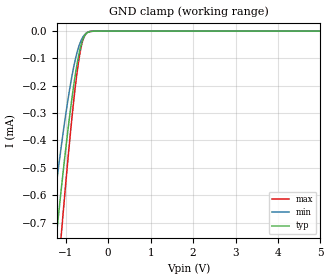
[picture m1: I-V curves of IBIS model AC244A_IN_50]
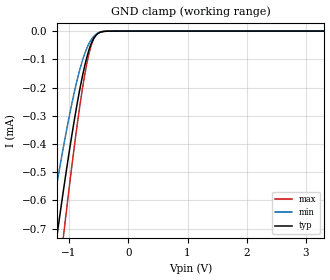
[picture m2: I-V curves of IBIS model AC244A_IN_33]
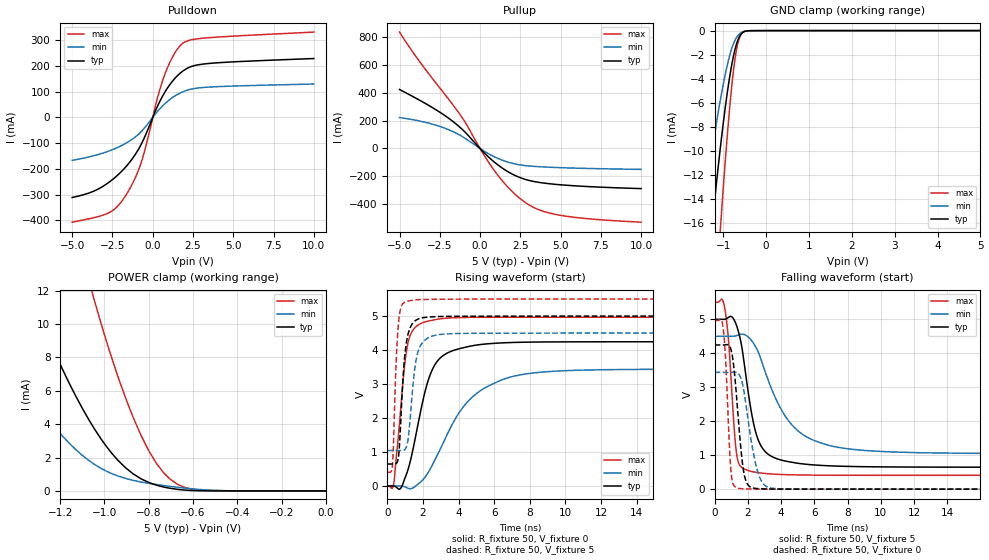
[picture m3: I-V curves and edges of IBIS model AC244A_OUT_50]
| TEXAS INSTRUMENTS INCORPORATED
| Standard Linear and Logic Group
| IBIS Model of SN74AC244
| OCTAL BUFFERS/DRIVERS WITH 3-STATE OUTPUTS
| This file contains package information for the following:
|  TSSOP 20-pin (PW) package as [Component] SN74AC244_PW
| This device can be powered at the following Vccs:
|  5 volt Vcc
|  3.3 volt Vcc
| This file provides unique models under the [Model Selector] for each Vcc.
| For operation at a specific Vcc, select the appropriate model after each
| [Model Selector] keyword.
[IBIS Ver]   3.2
[Comment char]  |_char
[File Name]   sn54ac244.ibs
[File Rev]   1.0 | a_die
[Date]   September 18, 2009
[Source]   Data created from TI-SPICE simulations at TI-SLL.
[Notes]   The following is an IBIS list for the SN74AC244.
   Please contact sllibis@ti.com with questions and
   comments concerning SLL IBIS models.
|   Modified from SN74 to SN54 devices with modified package
|   parasitics.   WVB 091809
[Disclaimer] Property of Texas Instruments Incorporated.  Unauthorized
   reproduction and/or distribution is strictly prohibited.
   This product is protected under copyright law.
   Created  2009, (C) Copyright  2009, Texas Instruments
   Incorporated, All Rights Reserved
   UNLESS THERE IS A SIGNED, WRITTEN AGREEMENT TO THE
   CONTRARY, TEXAS INSTRUMENTS (TI) IS PROVIDING THE IBIS
   MODELS  AND WITHOUT ANY WARRANTY, EXPRESSED OR
   IMPLIED.  TI assumes no liability for:
   1) the accuracy of the IBIS models provided to your
   company;
   2) the proper functioning of these IBIS Models in your
   design or for any resulting applications; or
   3) infringement of patents, copyrights or intellectual
   property rights resulting from your use of these IBIS
   models.
   TI provides IBIS Models as a service to our customers.
   You and your company shall not distribute, sell or give
   these models to anyone else without prior written
   permission from TI.
   TI reserves the right to make changes to our products or
   to discontinue any semiconductor product or service
   without notice, and advises our customers to obtain the
   latest version of relevant information to verify, before
   placing orders, that the information being relied on is
   current.
   Please be aware that your receipt and use of the IBIS
   information provided shall serve as acceptance of these
   terms and conditions.  If you do not accept these terms,
   you should return or destroy the IBIS models and any
   other accompanying information immediately.
| Component SN55AC244_W 20-PIN
[Component]   SN54AC244W
[Manufacturer]   Texas Instruments, Inc.
[Package]
|   typ   min   max
R_pkg   13.4e-02   9.30e-02   18.0e-02
L_pkg   6.136e-09   4.282e-09   8.371e-09
C_pkg   16.57e-13   12.24e-13   22.53e-13
[Pin]   signal_name   model_name   R_pin   L_pin   C_pin
1   N1OE   AC244A_OE   16.1e-2   8.173e-9   22.44e-13
2   1A1   AC244A_IN   16.3e-2   7.152e-9   20.34e-13
3   2Y4   AC244A_OUT   15.4e-2   6.346e-9   16.04e-13
4   1A2   AC244A_IN   9.3e-2   4.737e-9   12.72e-13
5   2Y3   AC244A_OUT   9.7e-2   4.297e-9   12.27e-13
6   1A3   AC244A_IN   9.6e-2   4.289e-9   12.26e-13
7   2Y2   AC244A_OUT   9.3e-2   4.759e-9   12.69e-13
8   1A4   AC244A_IN   14.3e-2   6.181e-9   15.54e-13
9   2Y1   AC244A_OUT   16.4e-2   7.085e-9   19.05e-13
10   GND   GND   17.5e-2   8.294e-9   22.33e-13
11   2A1   AC244A_IN   18.0e-2   8.371e-9   22.39e-13
12   1Y4   AC244A_OUT   15.5e-2   7.195e-9   19.34e-13
13   2A2   AC244A_IN   15.4e-2   6.339e-9   15.81e-13
14   1Y3   AC244A_OUT   9.6e-2   4.872e-9   12.81e-13
15   2A3   AC244A_IN   9.7e-2   4.338e-9   12.33e-13
16   1Y2   AC244A_OUT   9.7e-2   4.282e-9   12.24e-13
17   2A4   AC244A_IN   9.3e-2   4.726e-9   12.62e-13
18   1Y1   AC244A_OUT   14.3e-2   6.164e-9   15.71e-13
19   N2OE   AC244A_OE   15.9e-2   6.938e-9   20.01e-13
20   VCC   POWER   16.6e-2   8.186e-9   22.53e-13
| Component SN55AC244_J 20-PIN
[Component]   SN54AC244J
[Manufacturer]   Texas Instruments, Inc.
[Package]
|   typ   min   max
R_pkg   14.4e-02   9.70e-02   17.8e-02
L_pkg   18.08e-09   11.83e-09   25.95e-09
C_pkg   29.24e-13   16.25e-13   41.80e-13
[Pin]   signal_name   model_name   R_pin   L_pin   C_pin
1   N1OE   AC244A_OE   17.8e-02   25.95e-09   4.180e-12
2   1A1   AC244A_IN   16.7e-02   22.27e-09   3.807e-12
3   2Y4   AC244A_OUT   15.6e-02   17.47e-09   2.946e-12
4   1A2   AC244A_IN   12.1e-02   12.87e-09   2.062e-12
5   2Y3   AC244A_OUT   9.7e-02   11.83e-09   1.625e-12
6   1A3   AC244A_IN   9.7e-02   11.83e-09   1.625e-12
7   2Y2   AC244A_OUT   12.1e-02   12.87e-09   2.062e-12
8   1A4   AC244A_IN   15.6e-02   17.47e-09   2.946e-12
9   2Y1   AC244A_OUT   16.7e-02   22.27e-09   3.807e-12
10   GND   GND   17.8e-02   25.95e-09   4.180e-12
11   2A1   AC244A_IN   17.8e-02   25.95e-09   4.180e-12
12   1Y4   AC244A_OUT   16.7e-02   22.27e-09   3.807e-12
13   2A2   AC244A_IN   15.6e-02   17.47e-09   2.946e-12
14   1Y3   AC244A_OUT   12.1e-02   12.87e-09   2.062e-12
15   2A3   AC244A_IN   9.7e-02   11.83e-09   1.625e-12
16   1Y2   AC244A_OUT   9.7e-02   11.83e-09   1.625e-12
17   2A4   AC244A_IN   12.1e-02   12.87e-09   2.062e-12
18   1Y1   AC244A_OUT   15.6e-02   17.47e-09   2.946e-12
19   N2OE   AC244A_OE   16.7e-02   22.27e-09   3.807e-12
20   VCC   POWER   17.8e-02   25.95e-09   4.180e-12
| Component SN55AC244_FK 20-PIN
[Component]   SN54AC244FK
[Manufacturer]   Texas Instruments, Inc.
[Package]
|   typ   min   max
R_pkg   8.7e-02   8.20e-02   9.3e-02
L_pkg   3.13e-09   2.958e-09   3.28e-09
C_pkg   7.21e-13   6.59e-13   8.2e-13
[Pin]   signal_name   model_name   R_pin   L_pin   C_pin
1   N1OE   AC244A_OE   9.3e-02   3.226e-09   6.59e-13
2   1A1   AC244A_IN   8.2e-02   2.958e-09   7.17e-13
3   2Y4   AC244A_OUT   8.3e-02   3.163e-09   8.20e-13
4   1A2   AC244A_IN   8.4e-02   3.022e-09   7.26e-13
5   2Y3   AC244A_OUT   9.2e-02   3.280e-09   6.82e-13
6   1A3   AC244A_IN   9.3e-02   3.226e-09   6.59e-13
7   2Y2   AC244A_OUT   8.2e-02   2.958e-09   7.17e-13
8   1A4   AC244A_IN   8.3e-02   3.163e-09   8.20e-13
9   2Y1   AC244A_OUT   8.4e-02   3.022e-09   7.26e-13
10   GND   GND   9.2e-02   3.280e-09   6.82e-13
11   2A1   AC244A_IN   9.3e-02   3.226e-09   6.59e-13
12   1Y4   AC244A_OUT   8.2e-02   2.958e-09   7.17e-13
13   2A2   AC244A_IN   8.3e-02   3.163e-09   8.20e-13
14   1Y3   AC244A_OUT   8.4e-02   3.022e-09   7.26e-13
15   2A3   AC244A_IN   9.2e-02   3.280e-09   6.82e-13
16   1Y2   AC244A_OUT   9.3e-02   3.226e-09   6.59e-13
17   2A4   AC244A_IN   8.2e-02   2.958e-09   7.17e-13
18   1Y1   AC244A_OUT   8.3e-02   3.163e-09   8.20e-13
19   N2OE   AC244A_OE   8.4e-02   3.022e-09   7.26e-13
20   VCC   POWER   9.2e-02   3.280e-09   6.82e-13
| Model AC244A_IN
[Model Selector]   AC244A_IN
AC244A_IN_50   5 volt Vcc
AC244A_IN_33   3.3 volt Vcc
| Model AC244A_OE
[Model Selector]   AC244A_OE
AC244A_OE_50   5 volt Vcc
AC244A_OE_33   3.3 volt Vcc
| Model AC244A_OUT
[Model Selector]   AC244A_OUT
AC244A_OUT_50   5 volt Vcc
AC244A_OUT_33   3.3 volt Vcc
| Models and submodels in the file (6): AC244A_IN_50 (Input), AC244A_IN_33 (Input), AC244A_OE_50 (Input), AC244A_OE_33 (Input), AC244A_OUT_50 (3-state), AC244A_OUT_33 (3-state)
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[Model]   AC244A_IN_50
Model_type  Input
Vinl=1.35
Vinh=3.85
| variable   typ   min   max
C_comp   0.77pF   0.69pF   0.84pF
[Temperature Range]   40   100   -40
| Ambient temperature   25   85   -40
[Voltage range]   5   4.5   5.5
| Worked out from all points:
|   GND clamp passes 1 mA (typ) near -1.38 V on its own axis
[GND Clamp]
| AC244A_IN_50
|   Voltage   I(typ)   I(min)   I(max)
-5V       -7.834mA   -6.491mA   -8.926mA
-1.4V     -1.031mA   -788.3uA   -1.305mA
-1.345V   -943.5uA   -717uA     -1.198mA
-1.22V    -749.9uA   -559.7uA   -959.9uA
-1.195V   -712.2uA   -529.2uA   -913uA
-1.105V   -579.3uA   -422.4uA   -746.6uA
-1.08V    -543.4uA   -393.8uA   -701.3uA
-890mV    -289.7uA   -197.1uA   -375.4uA
-725mV    -114.1uA   -74.02uA   -143.2uA
-605mV    -34.41uA   -24.51uA   -38.71uA
-475mV    -4.506uA   -3.59uA    -3.661uA
5V        7.166nA    474.1pA    66.12nA
[Model]   AC244A_IN_33
Model_type  Input
Vinl=0.8
Vinh=2.0
| variable   typ   min   max
C_comp   0.78pF   0.70pF   0.85pF
[Temperature Range]   40   100   -40
| Ambient temperature   25   85   -40
[Voltage range]   3.3   3   3.6
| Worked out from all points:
|   GND clamp passes 1 mA (typ) near -1.38 V on its own axis
[GND Clamp]
| AC244A_IN_33
|   Voltage   I(typ)   I(min)   I(max)
-3.3V     -4.463mA   -3.643mA   -5.247mA
-1.365V   -975.1uA   -742.8uA   -1.237mA
-1.325V   -912uA     -691.3uA   -1.16mA
-1.205V   -727.2uA   -541.3uA   -931.7uA
-1.17V    -674.8uA   -499uA     -866.3uA
-1.08V    -543.4uA   -393.8uA   -701.3uA
-885mV    -283.6uA   -192.6uA   -367.4uA
-740mV    -127.5uA   -82.68uA   -160.9uA
-625mV    -43.98uA   -30.44uA   -50.86uA
-565mV    -19.84uA   -15.07uA   -20.7uA
-505mV    -7.613uA   -6.114uA   -6.771uA
3.3V      1.837nA    303.9pA    8.84nA
[Model]   AC244A_OUT_50
Model_type  3-state
Enable   Active-Low
Vref =   0
Rref =   500
Cref =   50p
Vmeas =   2.5
| variable   typ   min   max
C_comp   4.90pF   4.52pF   5.33pF
| C_pullup   10.57pF   5.33pF   16.48pF
| C_pulldown   6.78pF   5.20pF   8.81pF
| C_tri-state   4.90pF   4.52pF   5.33pF
[Temperature Range]   40   100   -40
| Ambient temperature   25   85   -40
[Voltage range]   5   4.5   5.5
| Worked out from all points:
|   slope of the pulldown table from 0 to 0.75 V, typ, clamps not added: 7.63 ohm
|   slope of the pullup table from 0 to 0.75 V, typ, clamps not added: 8.91 ohm
|   GND clamp passes 1 mA (typ) near -0.68 V on its own axis
|   POWER clamp passes 1 mA (typ) near -0.87 V on its own axis
|   rising waveform, R_fixture 50, V_fixture 0: 20-80 % time 1.16ns typ, 2.49ns min, 545ps max; typ from 0 V to 4.24 V
|   falling waveform, R_fixture 50, V_fixture 5: 20-80 % time 918ps typ, 2.17ns min, 416ps max; typ from 5 V to 0.647 V
|   rising waveform, R_fixture 50, V_fixture 5: 20-80 % time 329ps typ, 417ps min, 223ps max; typ from 0.647 V to 5 V
|   falling waveform, R_fixture 50, V_fixture 0: 20-80 % time 455ps typ, 688ps min, 274ps max; typ from 4.24 V to 0 V
[GND Clamp]
| AC244A_OUT_50
|   Voltage   I(typ)   I(min)   I(max)
-5V       -222.5mA   -143.7mA   -285.1mA
-1.52V    -26.4mA    -16.53mA   -42.46mA
-1.47V    -24.34mA   -15.2mA    -39.4mA
-1.265V   -16.42mA   -10.09mA   -27.28mA
-1.24V    -15.51mA   -9.508mA   -25.86mA
-1.07V    -9.809mA   -5.815mA   -16.63mA
-1.045V   -9.04mA    -5.319mA   -15.34mA
-890mV    -4.773mA   -2.626mA   -8.047mA
-780mV    -2.433mA   -1.261mA   -3.895mA
-680mV    -994.6uA   -511.5uA   -1.386mA
-560mV    -196uA     -120.9uA   -203.2uA
5V        69.38nA    25.6uA     649.7nA
[POWER Clamp]
| AC244A_OUT_50
|   Voltage   I(typ)   I(min)   I(max)
-5V       273.8mA    174.9mA    444.7mA
-1.6V     21.93mA    11.75mA    46.45mA
-1.34V    11.96mA    5.876mA    28mA
-1.19V    7.299mA    3.295mA    18.9mA
-1.07V    4.253mA    1.818mA    12.58mA
-1.045V   3.71mA     1.587mA    11.39mA
-940mV    1.847mA    897.9uA    6.879mA
-835mV    727.3uA    535.7uA    3.332mA
-765mV    343.7uA    382.3uA    1.643mA
-705mV    161.1uA    275.2uA    719.9uA
-580mV    12.93uA    96.2uA     61.64uA
0V        0A         0A         0A
[Pulldown]
| AC244A_OUT_50
|   Voltage   I(typ)   I(min)   I(max)
-5V       -311.7mA   -167mA     -407.7mA
-3.69V    -287.6mA   -149.5mA   -390.6mA
-2.685V   -250.7mA   -129.9mA   -369.7mA
-2.165V   -223.7mA   -116.4mA   -344.4mA
-1.61V    -187.7mA   -98.33mA   -297mA
-705mV    -103mA     -54.43mA   -173mA
290mV     42.96mA    23.01mA    75.33mA
745mV     97.69mA    53.03mA    166.5mA
1.295V    146.4mA    80.39mA    242.9mA
1.84V     179.2mA    98.95mA    287.4mA
3.395V    209.5mA    117.7mA    309.9mA
10V       229.3mA    130mA      332.2mA
[Pullup]
| AC244A_OUT_50
|   Voltage   I(typ)   I(min)   I(max)
-5V       424mA      222.1mA    836.6mA
-3.72V    344.9mA    196.7mA    619.6mA
-1.74V    199.2mA    124.2mA    322.5mA
-925mV    117.1mA    72.97mA    188.9mA
130mV     -15.94mA   -9.959mA   -25.24mA
895mV     -98.36mA   -59.77mA   -159.5mA
1.71V     -165.2mA   -96.95mA   -275.5mA
2.525V    -211mA     -118.7mA   -363.7mA
3.535V    -241.3mA   -130mA     -434.6mA
4.77V     -258.7mA   -136.9mA   -475.7mA
6.775V    -274.2mA   -143.7mA   -505.6mA
10V       -288.4mA   -150.3mA   -529.8mA
[Ramp]
| AC244A_OUT_50
| variable   typ   min   max
dV/dt_r   2.60/1.18E-09   2.11/2.51E-09   3.02/5.56E-10
dV/dt_f   2.66/9.30E-10   2.11/2.18E-09   3.11/4.31E-10
R_load = 50
[Rising Waveform]
| AC244A_OUT_50
R_fixture =   50
C_fixture =   0
L_fixture =   0
V_fixture =   0
V_fixture_min = 0
V_fixture_max = 0
|   Time   V(typ)   V(min)   V(max)
0s        170.7pV    330.8pV    68.43pV
360ps     -1.179mV   -85.06uV   91.07mV
920ps     140.5mV    -12.2mV    3.323V
1.145ns   465.4mV    -65.25mV   4.185V
1.99ns    2.503V     182.7mV    4.805V
2.515ns   3.416V     608.9mV    4.877V
3.17ns    3.853V     1.308V     4.93V
4.63ns    4.112V     2.546V     4.961V
6.79ns    4.218V     3.188V     4.965V
22.99ns   4.244V     3.437V     4.965V
[Falling Waveform]
| AC244A_OUT_50
R_fixture =   50
C_fixture =   0
L_fixture =   0
V_fixture =   5
V_fixture_min = 4.5
V_fixture_max = 5.5
|   Time   V(typ)   V(min)   V(max)
0s        5V         4.5V       5.5V
610ps     5V         4.5V       5.309V
835ps     5.058V     4.499V     4.368V
1.315ns   4.816V     4.521V     1.055V
1.895ns   3.277V     4.526V     569.9mV
2.415ns   1.774V     4.232V     501.4mV
2.98ns    1.137V     3.54V      465.7mV
4.445ns   808.6mV    2.01V      424.9mV
6.385ns   699.9mV    1.362V     411.9mV
22.99ns   646.8mV    1.046V     407.9mV
[Rising Waveform]
| AC244A_OUT_50
R_fixture =   50
C_fixture =   0
L_fixture =   0
V_fixture =   5
V_fixture_min = 4.5
V_fixture_max = 5.5
|   Time   V(typ)   V(min)   V(max)
0s        646.7mV    1.045V     407.9mV
285ps     647.1mV    1.045V     634.6mV
490ps     662.7mV    1.046V     3.642V
620ps     859mV      1.046V     4.774V
995ps     3.929V     1.082V     5.413V
1.17ns    4.489V     1.413V     5.442V
1.48ns    4.827V     3.194V     5.47V
1.675ns   4.899V     3.863V     5.479V
2.525ns   4.978V     4.414V     5.491V
22.99ns   5V         4.5V       5.5V
[Falling Waveform]
| AC244A_OUT_50
R_fixture =   50
C_fixture =   0
L_fixture =   0
V_fixture =   0
V_fixture_min = 0
V_fixture_max = 0
|   Time   V(typ)   V(min)   V(max)
0s        4.244V     3.437V     4.965V
510ps     4.243V     3.437V     4.741V
655ps     4.249V     3.437V     3.84V
965ps     4.131V     3.438V     621.1mV
1.29ns    2.877V     3.439V     48.76mV
1.62ns    980.1mV    3.197V     14mV
1.885ns   235.4mV    2.48V      7.552mV
2.54ns    18.27mV    599.5mV    2.351mV
3.255ns   4.837mV    45.95mV    1.244mV
22.99ns   371.2nV    6.591uV    3.296nV
